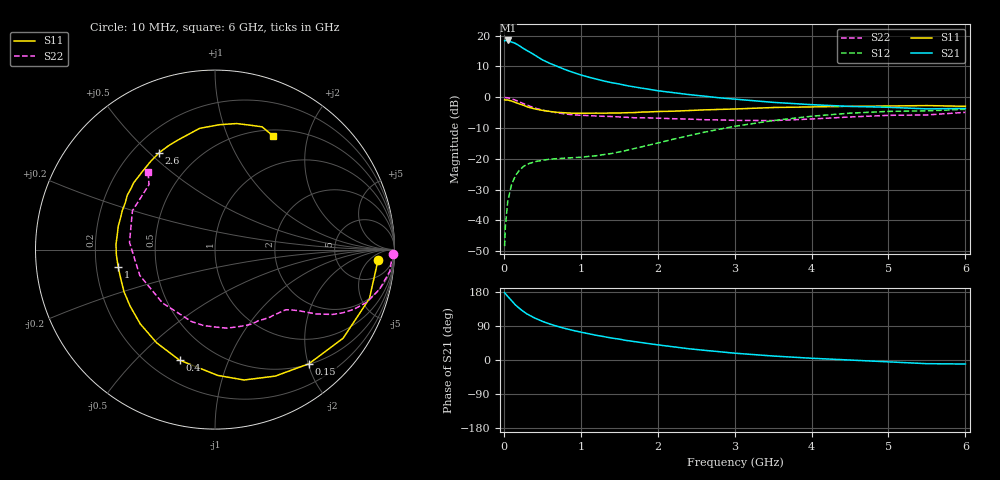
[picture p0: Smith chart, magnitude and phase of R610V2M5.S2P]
! SIEMENS Small Signal Semiconductors
! BFR193
! Si NPN RF Bipolar Junction Transistor in SOT23
! VCE = 10 V  IC = 2.5 mA
! Common Emitter S-Parameters:  May  1996
# GHz  S  MA  R  50
!  f  S11  S21  S12  S22
! GHz  MAG  ANG  MAG  ANG  MAG  ANG  MAG  ANG
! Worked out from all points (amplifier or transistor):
!   36 points, 10 MHz to 6 GHz, reference 50 ohm
!   highest |S21| = 18.5 dB at 50 MHz (marker M1)
!   |S21| within 3 dB of that: start of sweep to 282 MHz
!   unconditionally stable (mu >= 1): 1.127 GHz to 2.025 GHz
!   at 250 MHz: K = 0.26, MSG = 19.3 dB, |S12| = -22.6 dB
!   at 1.4 GHz: K = 1.09, MAG = 9.6 dB, |S12| = -18.3 dB
!   at 6 GHz: K = 0.98, MSG = 0.1 dB, |S12| = -3.9 dB
!   S11 on the Smith chart (normalised r, x): 10 MHz: 15, -10; 150 MHz: 0.51, -2.01; 400 MHz: 0.32, -0.68; 1 GHz: 0.29, -0.08; 2.6 GHz: 0.30, +0.54; 6 GHz: 0.57, +1.47
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0.01  0.91 -3.6  8.269 177.8  0.0038 84.2  0.9944 -1.3
0.02  0.9032 -7.2  8.354 175.0  0.0079 86.7  0.9865 -2.8
0.05  0.9027 -17.6  8.376 168.0  0.02 80.4  0.9814 -7.1
0.1  0.8679 -34.7  7.913 156.8  0.038 71.8  0.9441 -13.4
0.15  0.8234 -50.6  7.502 145.4  0.053 63.6  0.8968 -19.0
0.2  0.7808 -64.5  6.895 136.6  0.0647 57.0  0.842 -23.3
0.25  0.7444 -77.4  6.247 128.7  0.0741 51.9  0.7931 -26.4
0.3  0.701 -88.8  5.759 121.6  0.0813 48.0  0.7476 -28.9
0.4  0.647 -107.7  4.859 111.0  0.0894 42.4  0.6694 -32.4
0.5  0.6129 -122.0  4.064 102.1  0.0945 39.0  0.6172 -34.4
0.6  0.5872 -135.2  3.547 94.8  0.0986 37.3  0.5847 -35.8
0.7  0.5683 -146.3  3.155 88.5  0.1007 37.2  0.5574 -37.3
0.8  0.5587 -155.2  2.808 83.0  0.1024 37.8  0.5356 -38.8
1  0.5482 -170.0  2.305 73.6  0.1058 41.4  0.5101 -42.0
1.1  0.5504 -177.0  2.128 69.4  0.1093 43.4  0.503 -44.1
1.6  0.5607 156.9  1.543 51.4  0.1372 56.0  0.4723 -55.6
2.2  0.5932 133.5  1.19 34.9  0.2076 62.3  0.448 -73.9
2.6  0.6231 119.9  1.044 25.7  0.2693 60.6  0.4315 -89.5
3.5  0.6812 97.2  0.826 10.5  0.4174 47.0  0.4171 -134.4
4.5  0.7125 80.3  0.71 -0.1  0.5515 27.4  0.478 175.2
5.5  0.7326 69.0  0.647 -9.7  0.601 8.2  0.5157 135.5
6  0.712 63.2  0.658 -10.6  0.637 2.9  0.5686 130.9
